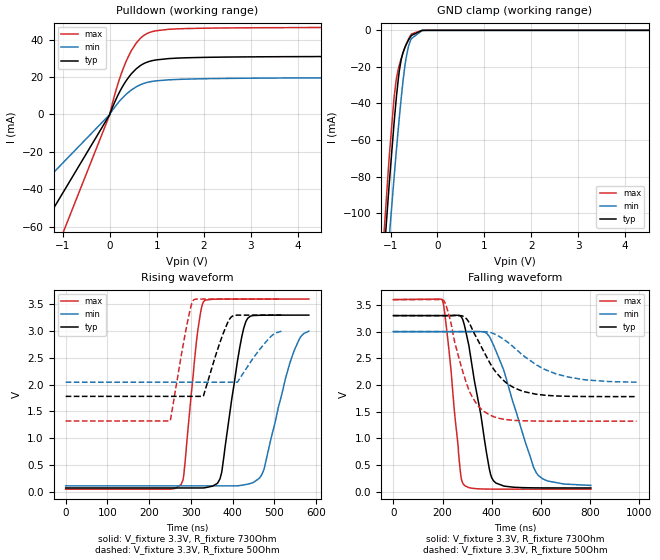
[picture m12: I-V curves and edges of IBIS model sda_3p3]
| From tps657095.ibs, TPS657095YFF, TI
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|   sda_3p3 Model
[Model]   sda_3p3
Model_type   I/O_open_drain
Polarity   Inverting
Vinl=0.4
Vinh=1.2
Vmeas = 1.65
Vref = 3.3
Cref = 400pF
Rref = 730
|   typ   min   max
|   (nom PVT)   (fast PVT)   (slow PVT)
C_comp   2.933e-12   2.933e-12   3.100e-12
| Where nom  PVT is Nominal Process, 3.3V, 27C
|   Fast PVT is Strong Process,  3.6V, -40C
|   Slow PVT is Weak Process,   3V, 125C
[Voltage Range]   3.3   3   3.6
|Junction Temperature
[Temperature Range]   27   125   -40
[Pullup Reference]   3.3   3   3.6
[Pulldown Reference]   0   0   0
[Power Clamp Reference]   3.3   3   3.6
[GND Clamp Reference]   0   0   0
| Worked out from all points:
|   slope of the pulldown table from 0 to 0.495 V, typ, clamps not added: 21.9 ohm
|   GND clamp passes 1 mA (typ) near -0.41 V on its own axis
|   falling waveform, V_fixture 3.3V, R_fixture 730Ohm: 20-80 % time 69.3ns typ, 118ns min, 44.1ns max; typ from 3.3 V to 0.07 V
|   rising waveform, V_fixture 3.3V, R_fixture 730Ohm: 20-80 % time 36.1ns typ, 54.8ns min, 26.2ns max; typ from 0.07 V to 3.3 V
|   falling waveform, V_fixture 3.3V, R_fixture 50Ohm: 20-80 % time 122ns typ, 180ns min, 86ns max; typ from 3.3 V to 1.78 V
|   rising waveform, V_fixture 3.3V, R_fixture 50Ohm: 20-80 % time 37.9ns typ, 53.7ns min, 30.7ns max; typ from 1.78 V to 3.3 V
[Pulldown]
|   Voltage   I(typ)   I(min)   I(max)
-3.3V     -138.2mA   -85.45mA   -209.3mA
-9mV      -376.8uA   -233uA     -570.9uA
161.7mV   9.708mA    5.74mA     15.45mA
260.7mV   14.45mA    8.593mA    22.88mA
359.7mV   18.43mA    11.02mA    29.06mA
462mV     21.79mA    13.1mA     34.2mA
562.8mV   24.38mA    14.73mA    38.11mA
688.8mV   26.69mA    16.24mA    41.5mA
789.6mV   27.89mA    17.06mA    43.17mA
987mV     29.12mA    17.93mA    44.71mA
1.647V    30.27mA    18.86mA    45.89mA
6.6V      31.11mA    19.69mA    46.66mA
[GND Clamp]
|   Voltage   I(typ)   I(min)   I(max)
-3.3V     -1.008A    -964.3mA   -1.067A
-1.201V   -145.4mA   -171.2mA   -134.7mA
-1.046V   -90.4mA    -119.4mA   -75.93mA
-1.023V   -82.44mA   -111.8mA   -67.63mA
-927.3mV  -51.53mA   -81.41mA   -37.5mA
-873.6mV  -36.14mA   -65.15mA   -26.19mA
-808.8mV  -21.47mA   -46.63mA   -18.55mA
-735mV    -12.24mA   -27.96mA   -12.41mA
-672mV    -8.096mA   -15.63mA   -7.973mA
-552mV    -2.772mA   -4.461mA   -1.979mA
-240mV    -2.402uA   -29.4uA    -383.3nA
6.6V      0A         101.8nA    0A
[POWER Clamp]
|   Voltage   I(typ)   I(min)   I(max)
-3.3V     0A         0A         0A
0V        0A         0A         0A
6.6V      0A         0A         0A
[Ramp]
R_load = 730
|   typ   min   max
dV/dt_r   1.93779/3.61752e-08   1.73421/5.47799e-08   2.13138/2.62717e-08
dV/dt_f   1.93779/6.90507e-08   1.73389/1.17622e-07   2.13138/4.40223e-08
[Falling Waveform]
V_fixture = 3.3V
V_fixture_min = 3V
V_fixture_max = 3.6V
R_fixture = 730Ohm
|   Time   V(typ)   V(min)   V(max)
0s        3.3V       3V         3.6V
200.2ns   3.3V       3V         3.578V
225.7ns   3.3V       3V         2.678V
274ns     3.288V     3V         323.9mV
288.8ns   3.124V     3V         121.2mV
390.5ns   425.7mV    2.908V     49.12mV
408ns     201.7mV    2.739V     48.5mV
581.1ns   72.2mV     355.8mV    47.71mV
626.9ns   71.04mV    201mV      47.71mV
803.1ns   70.37mV    118mV      47.71mV
[Rising Waveform]
V_fixture = 3.3V
V_fixture_min = 3V
V_fixture_max = 3.6V
R_fixture = 730Ohm
|   Time   V(typ)   V(min)   V(max)
0s        70.35mV    109.6mV    47.71mV
276.3ns   70.35mV    109.6mV    132.7mV
323.2ns   70.35mV    109.6mV    3.341V
363ns     152.5mV    109.6mV    3.598V
373.9ns   358.1mV    109.6mV    3.599V
422.2ns   2.897V     120.7mV    3.6V
450.2ns   3.292V     174.3mV    3.6V
474.9ns   3.298V     405.8mV    3.6V
547.9ns   3.3V       2.64V      3.6V
583ns     3.3V       3V         3.6V
[Falling Waveform]
V_fixture = 3.3V
V_fixture_min = 3V
V_fixture_max = 3.6V
R_fixture = 50Ohm
|   Time   V(typ)   V(min)   V(max)
0s        3.3V       3V         3.6V
204.7ns   3.3V       3V         3.583V
229.8ns   3.3V       3V         3.248V
278ns     3.297V     3V         2.318V
309.8ns   3.154V     3V         1.877V
393.9ns   2.401V     2.986V     1.435V
454ns     2.061V     2.839V     1.354V
534.1ns   1.872V     2.531V     1.328V
711ns     1.788V     2.15V      1.322V
988.6ns   1.782V     2.052V     1.322V
[Rising Waveform]
V_fixture = 3.3V
V_fixture_min = 3V
V_fixture_max = 3.6V
R_fixture = 50Ohm
|   Time   V(typ)   V(min)   V(max)
0s        1.782V     2.046V     1.322V
250.4ns   1.782V     2.046V     1.322V
290.1ns   1.782V     2.046V     3.098V
307.8ns   1.782V     2.046V     3.589V
330.2ns   1.79V      2.046V     3.6V
369.4ns   2.779V     2.046V     3.6V
395.8ns   3.256V     2.046V     3.6V
412.5ns   3.299V     2.055V     3.6V
478ns     3.3V       2.782V     3.6V
517.1ns   3.3V       3V         3.6V
